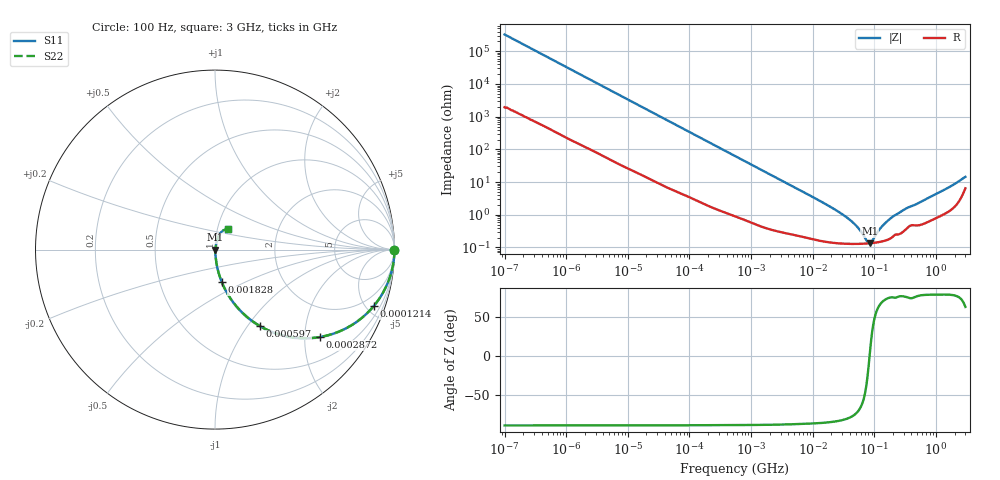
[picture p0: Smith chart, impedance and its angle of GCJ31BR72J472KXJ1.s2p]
!Murata Part Number: GCJ31BR72J472KXJ1
!These Parameters are Measured in Series Mode Connection
!Data Generated on Mar 13, 2026
!  o--ll--o
!Port1  Port2
!  o------o
!Operation Temp=25[degC], DC Bias Voltage=0[V]
!Freq. Start=100[Hz] Stop=3[GHz] 401[Steps]
# Hz S RI R 50
!Freq.(Hz) S11(Real) S11(Imag) S21(Real) S21(Imag) S12(Real) S12(Imag) S22(Real) S22(Imag)
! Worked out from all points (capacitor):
!   401 points, 100 Hz to 3 GHz, reference 50 ohm
!   read as one part in series: C = 4.85 nF near 109 Hz
!   lowest |Z| = 134 mohm at 84.26 MHz (marker M1)
!   series resonance near 83.59 MHz, so ESL is about 750 pH
!   S11 on the Smith chart (normalised r, x): 100 Hz: open; 121.4 kHz: 1.06, -5.59; 287.2 kHz: 1.03, -2.38; 597 kHz: 1.02, -1.15; 1.828 MHz: 1.01, -0.38; 3 GHz: 1.13, +0.26
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100  1 -0.000305  1.9e-06 0.000305  1.9e-06 0.000305  1 -0.000305
1788  0.9999 -0.00538  6.75e-05 0.00538  6.75e-05 0.00538  0.9999 -0.00538
31977  0.9903 -0.0939  0.00971 0.0939  0.00971 0.0939  0.9903 -0.0939
121426  0.884 -0.3151  0.116 0.3151  0.116 0.3151  0.884 -0.3151
186741  0.766 -0.4179  0.234 0.4179  0.234 0.4179  0.766 -0.4179
287190  0.5842 -0.4869  0.4158 0.4869  0.4158 0.4869  0.5842 -0.4869
547723  0.2842 -0.4439  0.7158 0.4439  0.7158 0.4439  0.2842 -0.4439
596961  0.2514 -0.4265  0.7486 0.4265  0.7486 0.4265  0.2514 -0.4265
1000599  0.11 -0.3047  0.89 0.3047  0.89 0.3047  0.11 -0.3047
1827928  0.038 -0.1814  0.962 0.1814  0.962 0.1814  0.038 -0.1814
9794414  0.00305 -0.0354  0.997 0.0354  0.997 0.0354  0.00305 -0.0354
2.316512e7  0.00156 -0.0142  0.9984 0.0142  0.9984 0.0142  0.00156 -0.0142
3.882828e7  0.00133 -0.00719  0.9987 0.00719  0.9987 0.00719  0.00133 -0.00719
5.478864e7  0.00129 -0.00371  0.9987 0.00371  0.9987 0.00371  0.00129 -0.00371
7.730952e7  0.00132 -0.000665  0.9987 0.000665  0.9987 0.000665  0.00132 -0.000665
8.425944e7  0.00134 6.96e-05  0.9987 -6.96e-05  0.9987 -6.96e-05  0.00134 6.96e-05
9.183415e7  0.00136 0.000805  0.9986 -0.000805  0.9986 -0.000805  0.00136 0.000805
1.295826e8  0.00152 0.00387  0.9985 -0.00387  0.9985 -0.00387  0.00152 0.00387
1.751444e8  0.00185 0.00696  0.9981 -0.00696  0.9981 -0.00696  0.00185 0.00696
3.199599e8  0.00369 0.0147  0.9963 -0.0147  0.9963 -0.0147  0.00369 0.0147
1.71441e9  0.0184 0.0697  0.9816 -0.0697  0.9816 -0.0697  0.0184 0.0697
3e9  0.0739 0.1123  0.9261 -0.1123  0.9261 -0.1123  0.0739 0.1123
